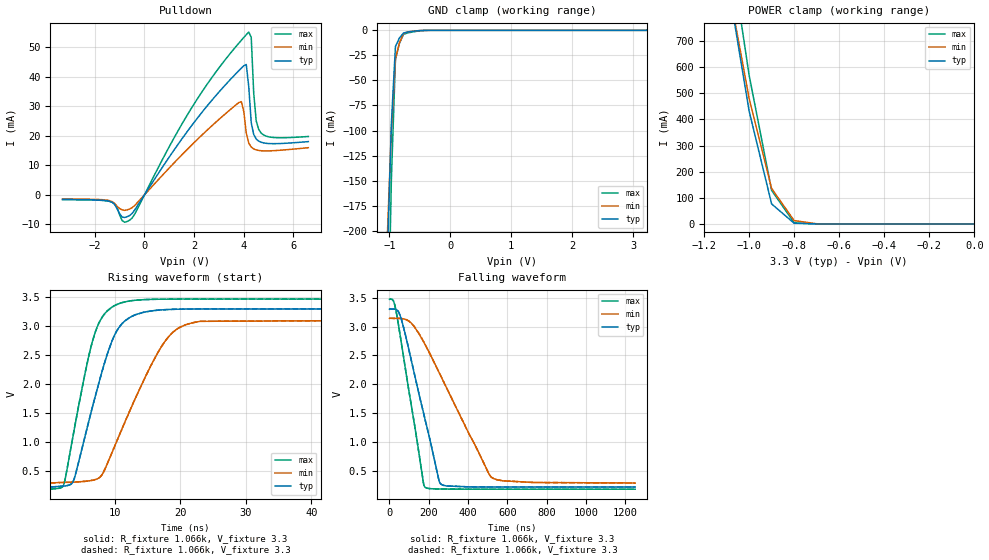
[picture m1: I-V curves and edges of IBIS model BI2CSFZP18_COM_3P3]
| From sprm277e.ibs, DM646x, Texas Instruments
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|   Model Cell BI2CSFZP18_COM_3P3
[Model]   BI2CSFZP18_COM_3P3
Model_type   I/O_open_drain
Polarity   Non-Inverting
Enable   Active-Low
Vinl =  0.99
Vinh =  2.31
Cref =  400pF
Rref =  1.066k
Vref =  1.8V
Vmeas =  1.65
C_comp   1.488594p   1.343646p   1.625598p
[Model Spec]
Vinl   0.99   0.942   1.041
Vinh   2.31   2.198   2.429
[Temperature Range]   25   105   0
[Voltage Range]   3.3   3.14   3.47
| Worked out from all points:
|   slope of the pulldown table from 0 to 0.495 V, typ, clamps not added: 76.9 ohm
|   GND clamp passes 1 mA (typ) near -0.62 V on its own axis
|   POWER clamp passes 1 mA (typ) near -0.73 V on its own axis
|   rising waveform, R_fixture 1.066k, V_fixture 3.3: 20-80 % time 4.48ns typ, 6.97ns min, 3.57ns max; typ from 0.221 V to 3.3 V
|   rising waveform, R_fixture 1.066k, V_fixture 3.3: 20-80 % time 4.48ns typ, 6.97ns min, 3.57ns max; typ from 0.221 V to 3.3 V
|   falling waveform, R_fixture 1.066k, V_fixture 3.3: 20-80 % time 126ns typ, 249ns min, 92.4ns max; typ from 3.3 V to 0.221 V
|   falling waveform, R_fixture 1.066k, V_fixture 3.3: 20-80 % time 126ns typ, 249ns min, 92.4ns max; typ from 3.3 V to 0.221 V
[POWER_clamp]
|   voltage   I(typ)   I(min)   I(max)
-3.3V     15.05A     13.75A     15.99A
-1.067V   781.2mA    793mA      954.4mA
-1.033V   606.9mA    637.3mA    762.2mA
-1V       432.7mA    481.5mA    570mA
-900mV    76.75mA    135.8mA    128.5mA
-800mV    2.774mA    12.97mA    4.49mA
-700mV    66.53uA    739.3uA    77.17uA
0V        40.21nA    28.69nA    188.6nA
[Pulldown]
|   voltage   I(typ)   I(min)   I(max)
-3.3V     -1.585mA   -1.413mA   -1.619mA
-1.4V     -2.214mA   -1.997mA   -2.244mA
-500mV    -6.316mA   -4.377mA   -7.884mA
1.8V      22.32mA    16.03mA    28.1mA
3.8V      42.06mA    31.25mA    51.39mA
4V        43.73mA    28.23mA    53.32mA
4.1V      44.15mA    20.94mA    54.26mA
4.2V      36.62mA    17.54mA    55.14mA
4.3V      24.45mA    16.18mA    53.34mA
4.4V      20.43mA    15.54mA    34.42mA
4.6V      18.2mA     15.03mA    22.16mA
6.6V      18.02mA    15.96mA    19.76mA
[GND_clamp]
|   voltage   I(typ)   I(min)   I(max)
-3.3V     -17.3A     -15.81A    -18.24A
-1.033V   -228.3mA   -206mA     -345.7mA
-966.7mV  -93.1mA    -99.19mA   -148.6mA
-900mV    -16.17mA   -28.6mA    -29.03mA
-833.3mV  -7.484mA   -12.28mA   -12.72mA
-766.7mV  -2.666mA   -3.264mA   -3.923mA
-700mV    -1.72mA    -1.56mA    -2.645mA
-633.3mV  -1.119mA   -1.016mA   -1.818mA
-366.7mV  -16.93uA   -31.45uA   -52.75uA
3.233V    39.65nA    29.26nA    179.4nA
[Ramp]
| variable   typ   min   max
dV/dt_f   1.73396/0.13001457u  1.5649288/0.25579991u  1.8779024/94.662309n
dV/dt_r 13.915375m/1.0960774n 8.8595326m/2.3934337n 16.515116m/0.78342627n
R_load = 528
[Rising Waveform]
R_fixture = 1.066k
V_fixture = 3.3
V_fixture_min = 3.14
V_fixture_max = 3.47
|   time   V(typ)   V(min)   V(max)
156.3ps   220.8mV    289.7mV    183.5mV
2.175ns   236.3mV    299.5mV    251.2mV
3.643ns   315.8mV    305.3mV    1.111V
6.215ns   1.438V     329.5mV    2.574V
7.795ns   2.113V     398.5mV    3.103V
10.89ns   3.017V     1.171V     3.401V
15.56ns   3.265V     2.332V     3.464V
18.85ns   3.292V     2.894V     3.469V
23.03ns   3.299V     3.085V     3.47V
1.25us    3.3V       3.14V      3.47V
[Rising Waveform]
R_fixture = 1.066k
V_fixture = 3.3
V_fixture_min = 3.14
V_fixture_max = 3.47
|   time   V(typ)   V(min)   V(max)
156.3ps   220.8mV    289.7mV    183.5mV
2.175ns   236.3mV    299.5mV    251.2mV
3.643ns   315.8mV    305.3mV    1.111V
6.215ns   1.438V     329.5mV    2.574V
7.795ns   2.113V     398.5mV    3.103V
10.89ns   3.017V     1.171V     3.401V
15.56ns   3.265V     2.332V     3.464V
18.85ns   3.292V     2.894V     3.469V
23.03ns   3.299V     3.085V     3.47V
1.25us    3.3V       3.14V      3.47V
[Falling Waveform]
R_fixture = 1.066k
V_fixture = 3.3
V_fixture_min = 3.14
V_fixture_max = 3.47
|   time   V(typ)   V(min)   V(max)
156.3ps   3.3V       3.14V      3.47V
25.97ns   3.301V     3.141V     3.388V
57.45ns   3.159V     3.138V     2.788V
113.6ns   2.381V     3.05V      1.591V
173.3ns   1.507V     2.74V      289.2mV
182.4ns   1.375V     2.682V     214.6mV
251.6ns   344.2mV    2.213V     186.4mV
260.9ns   274.1mV    2.147V     185.9mV
522.4ns   221mV      380.9mV    183.5mV
1.25us    220.8mV    289.7mV    183.5mV
[Falling Waveform]
R_fixture = 1.066k
V_fixture = 3.3
V_fixture_min = 3.14
V_fixture_max = 3.47
|   time   V(typ)   V(min)   V(max)
156.3ps   3.3V       3.14V      3.47V
25.97ns   3.301V     3.141V     3.388V
57.45ns   3.159V     3.138V     2.788V
113.6ns   2.381V     3.05V      1.591V
173.3ns   1.507V     2.74V      289.2mV
182.4ns   1.375V     2.682V     214.6mV
251.6ns   344.2mV    2.213V     186.4mV
260.9ns   274.1mV    2.147V     185.9mV
522.4ns   221mV      380.9mV    183.5mV
1.25us    220.8mV    289.7mV    183.5mV
